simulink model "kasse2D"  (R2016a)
settings: Solver=ode45  StartTime=0.0  StopTime=100  FixedStep=0.001  MaxStep=2  RelTol=1e-3
undefined symbols (not defined in the file or in its folder): tAb, z0
libraries: simulink x3

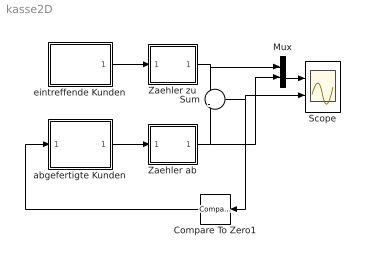
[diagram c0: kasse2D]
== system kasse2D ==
  Compare To Zero1 : simulink/Logic and Bit Operations/Compare To Zero  relop=<=  OutDataTypeStr=uint8
  Mux : Mux  Inputs=2
  Scope : Scope  NumInputPorts=2
  Sum : Sum  Inputs=+|-
  Zaehler ab : Subsystem
  Zaehler zu : Subsystem
  abgefertigte Kunden : Subsystem
  eintreffende Kunden : Subsystem
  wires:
  Zaehler zu/1(Out) -> Sum/1, Mux/1
  eintreffende Kunden/1(Out1) -> Zaehler zu/1(In)
  abgefertigte Kunden/1(Out) -> Zaehler ab/1(In)
  Zaehler ab/1(Out) -> Sum/2, Mux/2
  Sum/1 -> Compare To Zero1/1, Scope/2
  Compare To Zero1/1 -> abgefertigte Kunden/1(In1)
  Mux/1 -> Scope/1

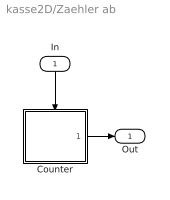
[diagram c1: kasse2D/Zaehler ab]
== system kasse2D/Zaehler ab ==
  In : Inport
  Counter : Subsystem
  Out : Outport
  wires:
  Counter/1(Out) -> Out/1
  In/1 -> Counter/Trigger

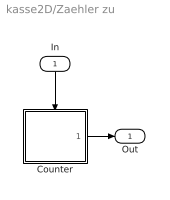
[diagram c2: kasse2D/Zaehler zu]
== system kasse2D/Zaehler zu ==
  In : Inport
  Counter : Subsystem
  Out : Outport
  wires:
  Counter/1(Out) -> Out/1
  In/1 -> Counter/Trigger

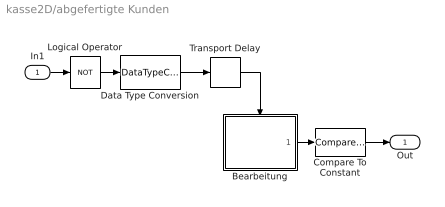
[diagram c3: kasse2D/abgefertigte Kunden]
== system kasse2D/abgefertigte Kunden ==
  In1 : Inport
  Bearbeitung : Subsystem
  Compare To Constant : simulink/Logic and Bit Operations/Compare To Constant  SystemSampleTime=-1  relop=>  const=tAb/2  LogicOutDataTypeMode=uint8
  Data Type Conversion : DataTypeConversion  OutDataTypeStr=double
  Logical Operator : Logic  Operator=NOT  AllPortsSameDT=off  OutDataTypeStr=boolean
  Transport Delay : TransportDelay  DelayTime=0.001*tAb
  Out : Outport
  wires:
  In1/1 -> Logical Operator/1
  Bearbeitung/1(Out1) -> Compare To Constant/1
  Logical Operator/1 -> Data Type Conversion/1
  Data Type Conversion/1 -> Transport Delay/1
  Transport Delay/1 -> Bearbeitung/Enable
  Compare To Constant/1 -> Out/1

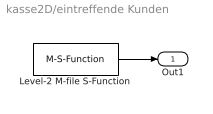
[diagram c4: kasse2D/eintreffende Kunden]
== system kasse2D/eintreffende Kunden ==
  Level-2 M-file S-Function : M-S-Function  FunctionName=sfun_poisson  Parameters=lambda
  Out1 : Outport
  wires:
  Level-2 M-file S-Function/1 -> Out1/1

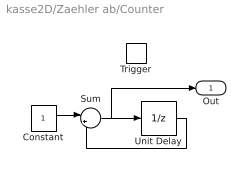
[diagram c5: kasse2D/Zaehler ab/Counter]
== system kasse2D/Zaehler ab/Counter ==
  Trigger : TriggerPort  TriggerType=falling  VariantControl=Variant
  Constant : Constant
  Sum : Sum  Inputs=|++
  Unit Delay : UnitDelay  InitialCondition=z0  SampleTime=-1
  Out : Outport  InitialOutput=z0
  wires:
  Constant/1 -> Sum/1
  Sum/1 -> Unit Delay/1, Out/1
  Unit Delay/1 -> Sum/2

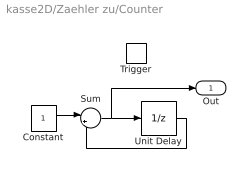
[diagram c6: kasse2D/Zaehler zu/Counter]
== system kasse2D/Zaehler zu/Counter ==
  Trigger : TriggerPort  TriggerType=falling  VariantControl=Variant
  Constant : Constant
  Sum : Sum  Inputs=|++
  Unit Delay : UnitDelay  InitialCondition=z0  SampleTime=-1
  Out : Outport  InitialOutput=z0
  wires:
  Constant/1 -> Sum/1
  Sum/1 -> Unit Delay/1, Out/1
  Unit Delay/1 -> Sum/2

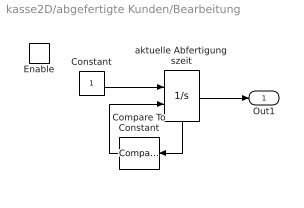
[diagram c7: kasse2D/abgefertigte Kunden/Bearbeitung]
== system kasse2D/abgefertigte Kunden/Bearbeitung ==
  Enable : EnablePort  StatesWhenEnabling=reset
  Compare To Constant : simulink/Logic and Bit Operations/Compare To Constant  SystemSampleTime=-1  relop=>=  const=tAb  LogicOutDataTypeMode=boolean
  Constant : Constant
  aktuelle Abfertigungszeit : Integrator  ExternalReset=rising  ShowStatePort=on
  Out1 : Outport  OutputWhenDisabled=reset  InitialOutput=0
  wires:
  Compare To Constant/1 -> aktuelle Abfertigungszeit/2
  aktuelle Abfertigungszeit/1 -> Out1/1
  Constant/1 -> aktuelle Abfertigungszeit/1
  aktuelle Abfertigungszeit/State -> Compare To Constant/1
